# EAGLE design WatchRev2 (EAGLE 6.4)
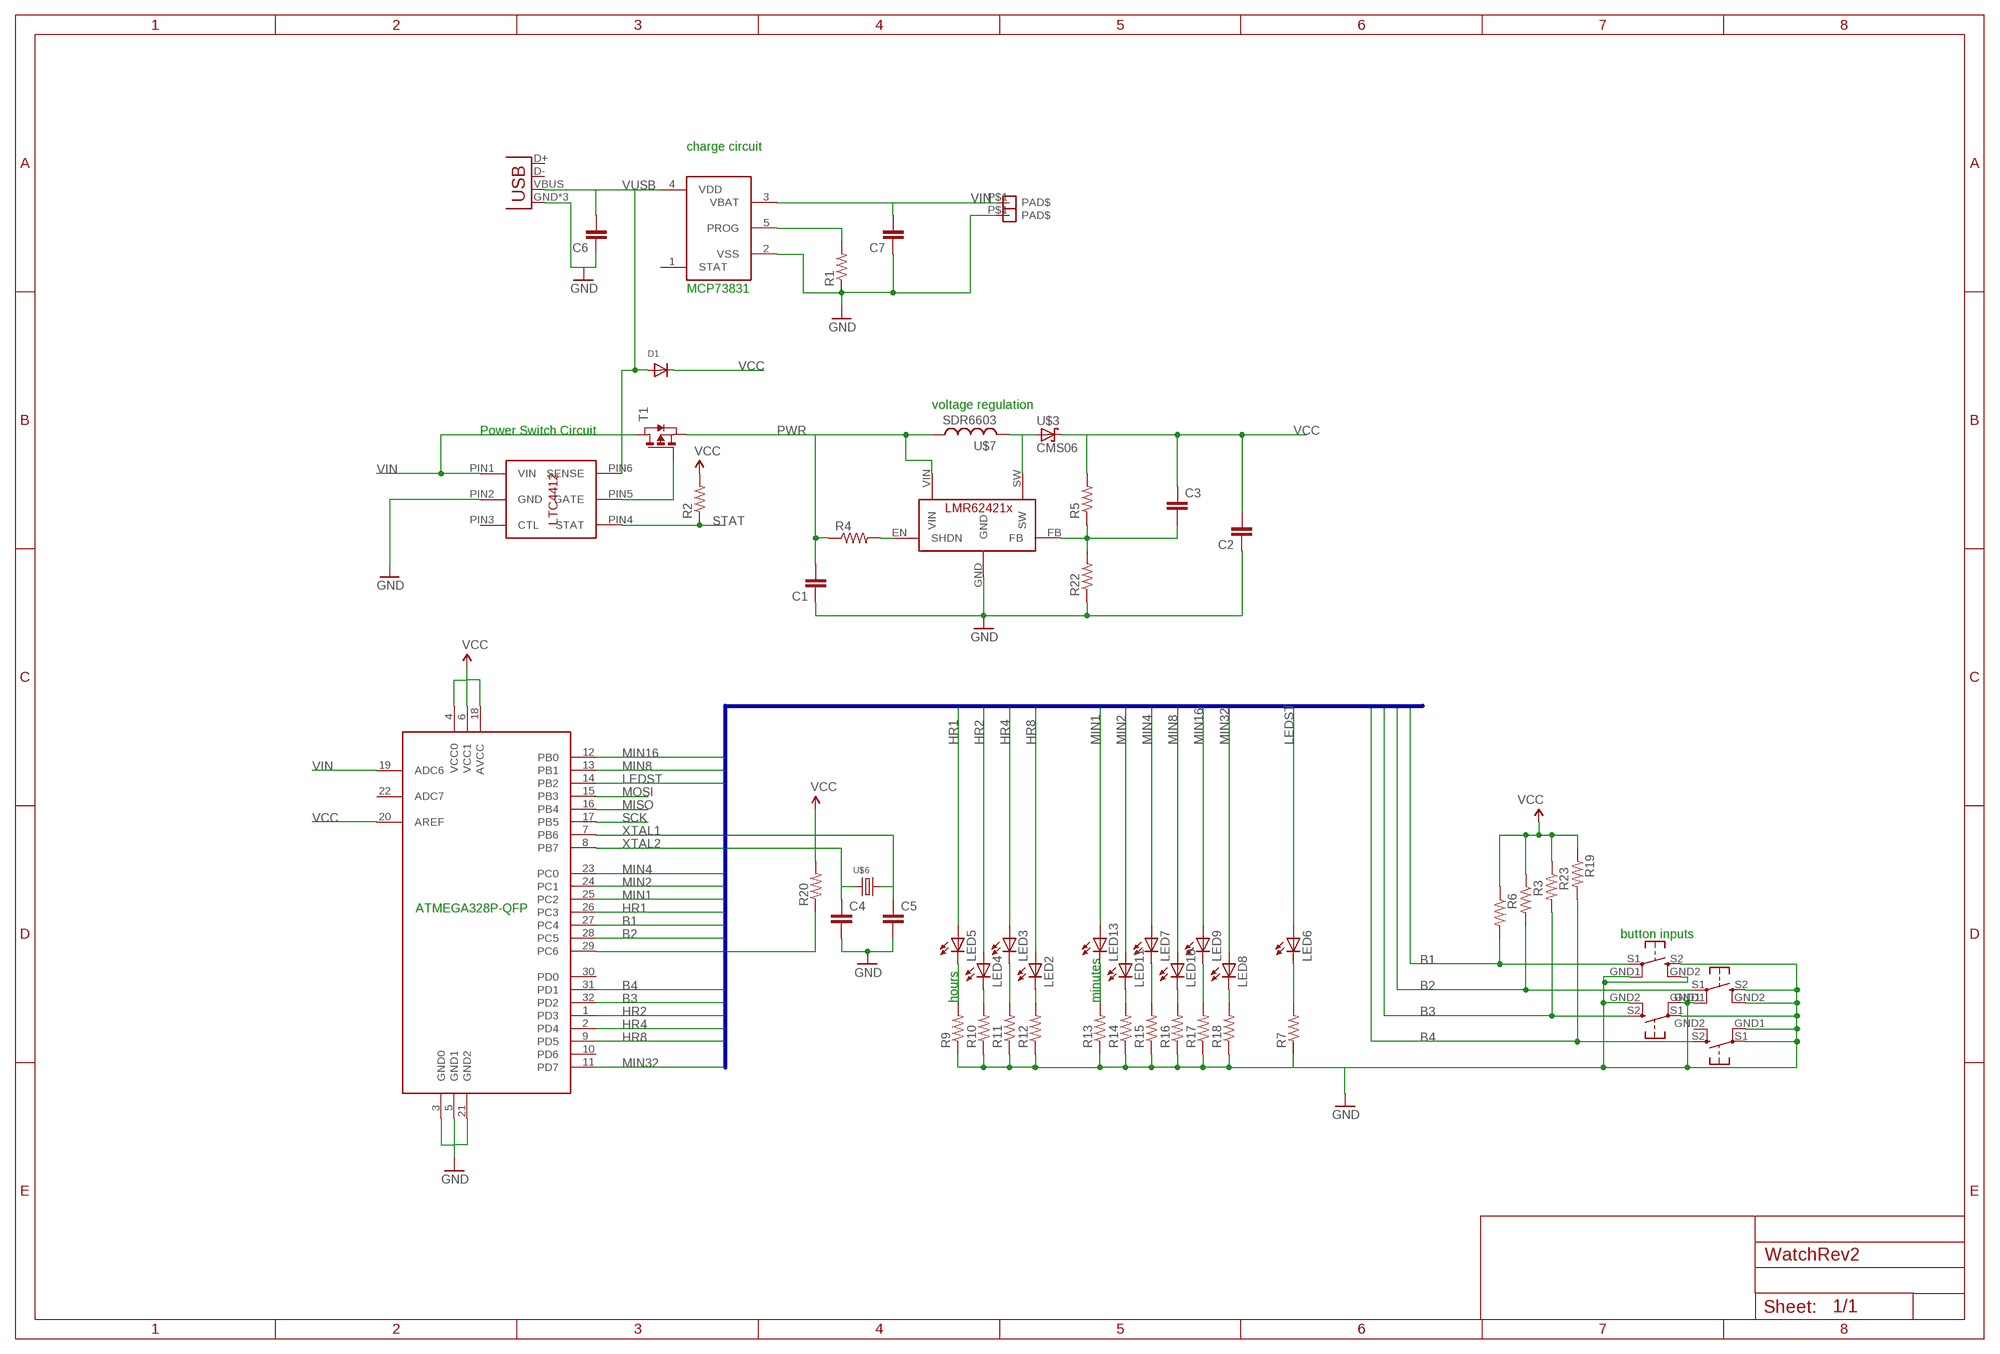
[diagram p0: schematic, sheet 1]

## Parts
C1  CAP0603-CAP  [0603-CAP]
C2  CAP0603-CAP  [0603-CAP]
C3  CAP0603-CAP  [0603-CAP]
C4  CAP0603-CAP  [0603-CAP]
C5  CAP0603-CAP  [0603-CAP]
C6  CAP0603-CAP  [0603-CAP]
C7  CAP0603-CAP  [0603-CAP]
D1  DIODESOD-123  [SOD-123]
JP5  USB-MICROB  [USB-MICROB]
LED2  LEDCHIPLED_1206  [CHIPLED_1206]
LED3  LEDCHIPLED_1206  [CHIPLED_1206]
LED4  LEDCHIPLED_1206  [CHIPLED_1206]
LED5  LEDCHIPLED_1206  [CHIPLED_1206]
LED6  LEDCHIPLED_0603  [CHIPLED_0603]
LED7  LEDCHIPLED_1206  [CHIPLED_1206]
LED8  LEDCHIPLED_1206  [CHIPLED_1206]
LED9  LEDCHIPLED_1206  [CHIPLED_1206]
LED10  LEDCHIPLED_1206  [CHIPLED_1206]
LED11  LEDCHIPLED_1206  [CHIPLED_1206]
LED13  LEDCHIPLED_1206  [CHIPLED_1206]
R1  RESISTOR0603-RES  [0603-RES]
R2  RESISTOR0603-RES  [0603-RES]
R3  RESISTOR0603-RES  [0603-RES]
R4  RESISTOR0603-RES  [0603-RES]
R5  RESISTOR0603-RES  [0603-RES]
R6  RESISTOR0603-RES  [0603-RES]
R7  RESISTOR0603-RES  [0603-RES]
R9  RESISTOR0603-RES  [0603-RES]
R10  RESISTOR0603-RES  [0603-RES]
R11  RESISTOR0603-RES  [0603-RES]
R12  RESISTOR0603-RES  [0603-RES]
R13  RESISTOR0603-RES  [0603-RES]
R14  RESISTOR0603-RES  [0603-RES]
R15  RESISTOR0603-RES  [0603-RES]
R16  RESISTOR0603-RES  [0603-RES]
R17  RESISTOR0603-RES  [0603-RES]
R18  RESISTOR0603-RES  [0603-RES]
R19  RESISTOR0603-RES  [0603-RES]
R20  RESISTOR0603-RES  [0603-RES]
R22  RESISTOR0603-RES  [0603-RES]
R23  RESISTOR0603-RES  [0603-RES]
T1  PMOSSOT23  [SOT-23]
U$1  ATMEGA328P  [TQFP32-08]
U$2  LMR62421X  [SOT-23_5PIN]
U$3  CMS06  [SOD-128]
U$4  MCP73831  [SOT-23_5GEN]
U$5  LTC4412  [LTC4412]
U$6  ECX-39  [ECX-39]
U$7  SDR6603  [SDR6603]
U$8  PAD  [PAD]
U$9  PAD  [PAD]
U$10  RA_TAC_BUTTON  [RA_TAC_BUTTON]
U$11  RA_TAC_BUTTON  [RA_TAC_BUTTON]
U$12  RA_TAC_BUTTON  [RA_TAC_BUTTON]
U$13  RA_TAC_BUTTON  [RA_TAC_BUTTON]

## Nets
B1: R6.2 U$1.27(PC4) U$10.S1
B2: R3.2 U$1.28(PC5) U$11.S1
B3: R23.2 U$1.32(PD2) U$12.S2
B4: R19.2 U$1.31(PD1) U$13.S2
GND: C1.1 C2.1 C4.2 C5.2 C6.1 C7.1 JP5.GND JP5.MT1(GND) JP5.MT2(GND) R1.1 R7.1 R9.1 R10.1 R11.1 R12.1 R13.1 R14.1 R15.1 R16.1 R17.1 R18.1 R22.1 U$1.3(GND0) U$1.5(GND1) U$1.21(GND2) U$2.GND U$4.2(VSS) U$5.PIN2(GND) U$9.P$1(PAD$) U$10.GND1 U$10.GND2 U$10.S2 U$11.GND1 U$11.GND2 U$11.S2 U$12.GND1 U$12.GND2 U$12.S1 U$13.GND1 U$13.S1
HR1: LED5.A U$1.26(PC3)
HR2: LED4.A U$1.1(PD3)
HR4: LED3.A U$1.2(PD4)
HR8: LED2.A U$1.9(PD5)
LEDST: LED6.A U$1.14(PB2)
MIN1: LED13.A U$1.25(PC2)
MIN2: LED11.A U$1.24(PC1)
MIN4: LED7.A U$1.23(PC0)
MIN8: LED10.A U$1.13(PB1)
MIN16: LED9.A U$1.12(PB0)
MIN32: LED8.A U$1.11(PD7)
MISO: U$1.16(PB4)
MOSI: U$1.15(PB3)
N$2: LED5.C R9.2
N$3: U$2.SW U$3.2(A) U$7.P$2
N$4: LED4.C R10.2
N$5: LED6.C R7.2
N$6: C3.2 R5.1 R22.2 U$2.FB
N$7: LED3.C R11.2
N$8: LED2.C R12.2
N$9: R4.2 U$2.EN(SHDN)
N$10: LED13.C R13.2
N$11: LED11.C R14.2
N$12: LED7.C R15.2
N$13: LED10.C R16.2
N$14: LED9.C R17.2
N$15: LED8.C R18.2
N$16: R20.1 U$1.29(PC6)
N$19: T1.3(G) U$5.PIN5(GATE)
N$21: R1.2 U$4.5(PROG)
PWR: C1.2 R4.1 T1.2(S) U$2.VIN U$7.P$1
SCK: U$1.17(PB5)
STAT: R2.1 U$5.PIN4(STAT)
VCC: C2.2 C3.1 D1.C R2.2 R3.1 R5.2 R6.1 R19.1 R20.2 R23.1 U$1.4(VCC0) U$1.6(VCC1) U$1.18(AVCC) U$1.20(AREF) U$3.1(C)
VIN: C7.2 T1.1(D) U$1.19(ADC6) U$4.3(VBAT) U$5.PIN1(VIN) U$8.P$1(PAD$)
VUSB: C6.2 D1.A JP5.VBUS U$4.4(VDD) U$5.PIN6(SENSE)
XTAL1: C5.1 U$1.7(PB6) U$6.P$2
XTAL2: C4.1 U$1.8(PB7) U$6.P$1
Unconnected: JP5.D+ JP5.D- U$1.10(PD6) U$1.22(ADC7) U$1.30(PD0) U$4.1(STAT) U$5.PIN3(CTL) U$13.GND2

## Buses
MIN32,MIN16,MIN8,MIN4,MIN2,MIN1,HR8,HR4,HR2,HR1,LEDST,B[1..4]

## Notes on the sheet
- charge circuit
- MCP73831
- voltage regulation
- Power Switch Circuit
- ATMEGA328P-QFP
- button inputs
- hours | minutes

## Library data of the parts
C1-C7 = SparkFun-Capacitors:CAP: Capacitor
D1 = adafruit:DIODE: Diode
JP5 = SparkFun-Connectors:USB: USB Connectors USB-B-PTH is fully proven SKU : PRT-00139/CONN-08278 USB-miniB is fully proven SKU : PRT-00587 USB-A-PCB is untested. USB-A-H is throughly reviewed, but untested. Spark Fun Electronics SKU : PRT-00437 USB-B-SMT is throughly reviewed, but untested. Needs silkscreen touching up.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; PROD_ID: CONN-09505
LED2-LED5 LED7-LED11 LED13 = adafruit:LED: LED
LED6 = led:LED: LED
R1-R7 R9-R20 R22 R23 = SparkFun-Passives:RESISTOR: Resistor
T1 = zetex:PMOSSOT23: MOS FET; OC_FARNELL: unknown; OC_NEWARK: unknown
U$1 = atmel:ATMEGA328P
U$2 = ubuntuMisc:LMR62421X
U$3 = ubuntuMisc:CMS06
U$4 = ubuntuMisc:MCP73831
U$5 = MyLibrary:LTC4412
U$6 = MyLibrary:ECX-39
U$7 = ubuntuMisc:SDR6603
U$8 U$9 = MyLibrary:PAD
U$10-U$13 = MyLibrary:RA_TAC_BUTTON

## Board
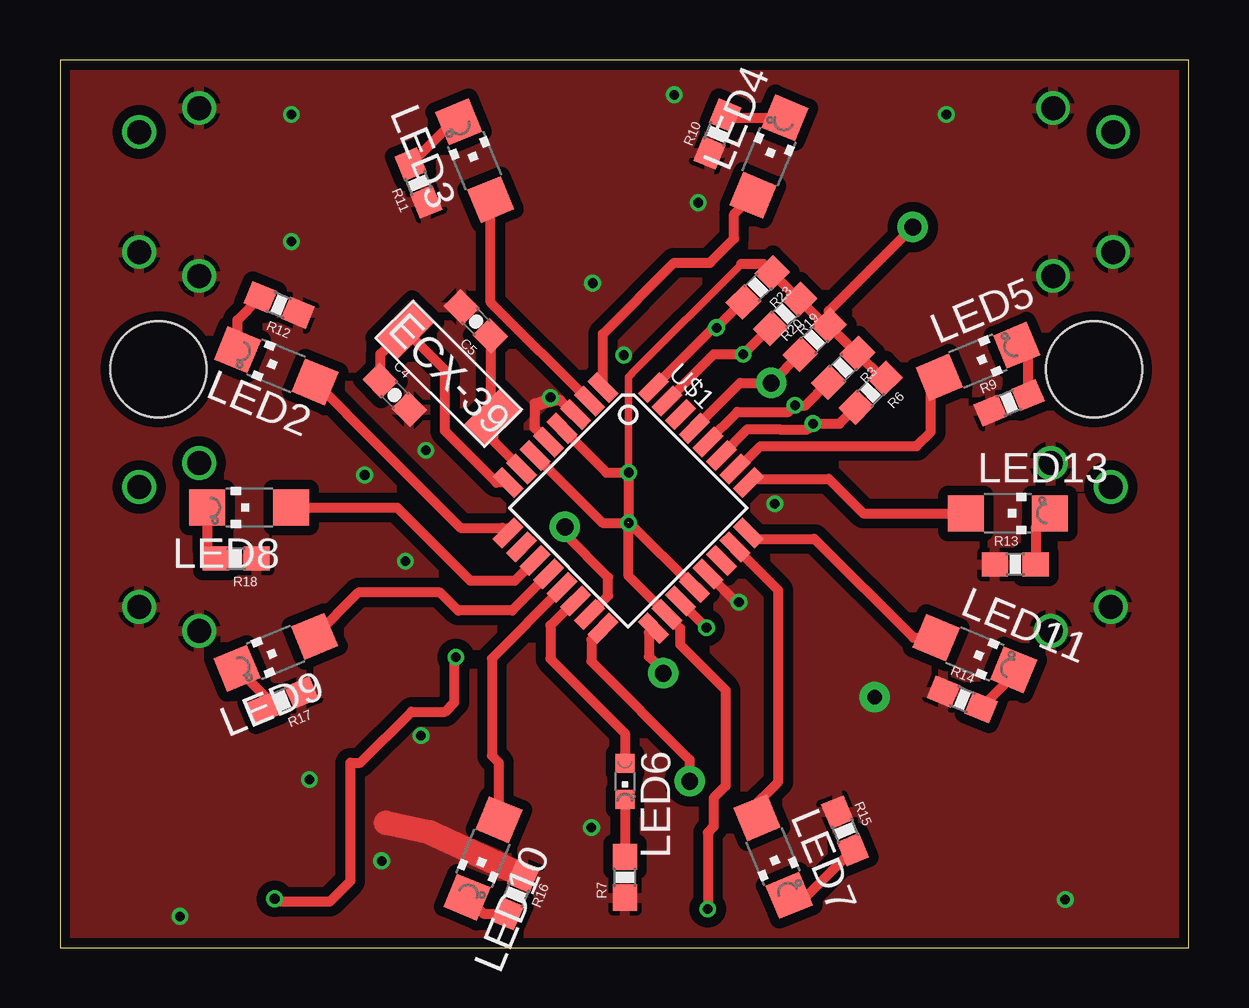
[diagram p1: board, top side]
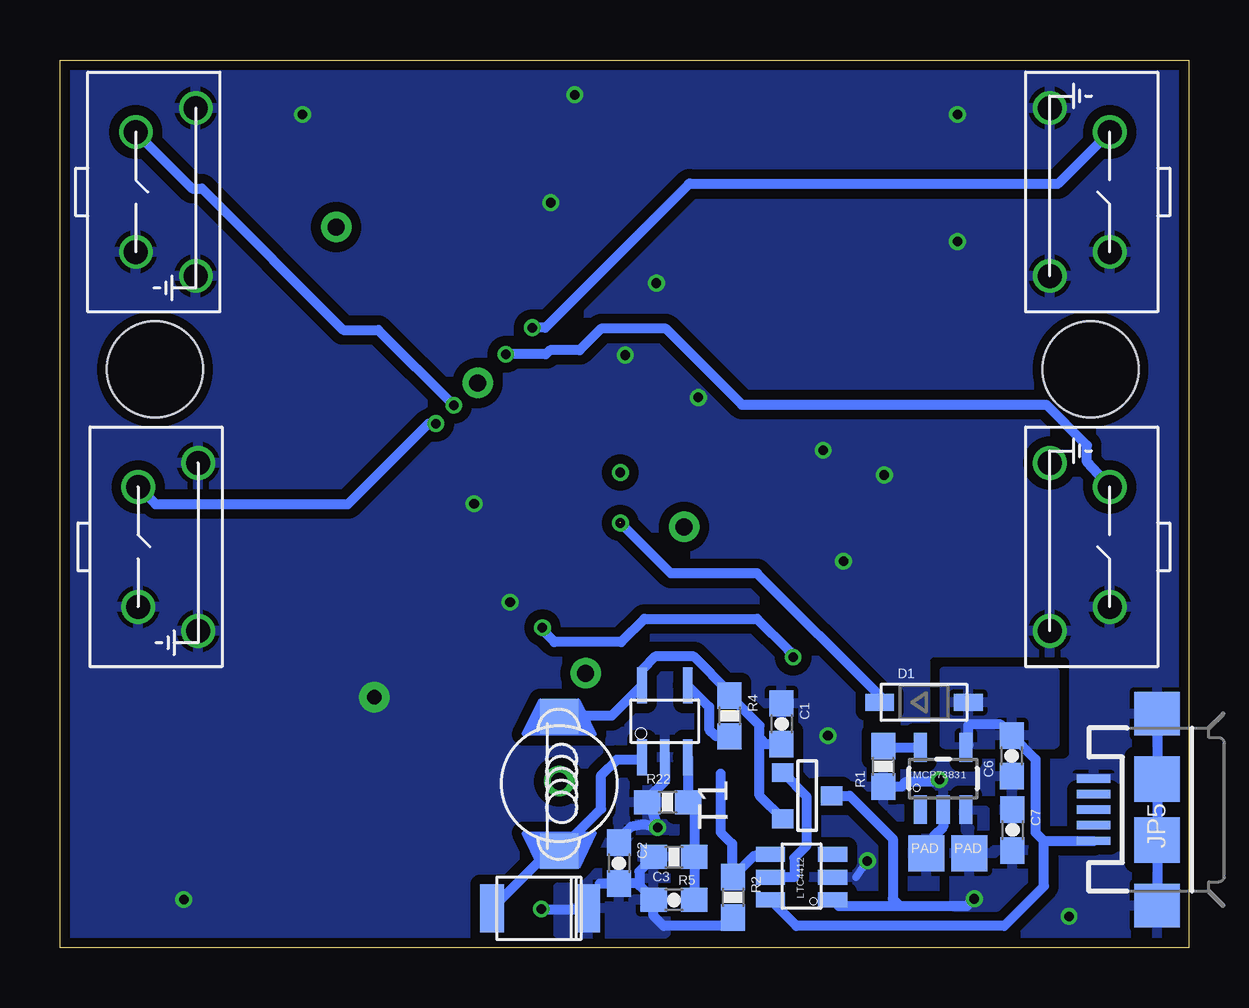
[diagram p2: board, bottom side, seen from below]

Size 47.06 x 37 mm. Coordinates in mm from the lower left corner, seen from the top.
Outline: 0,0 47.06,0 47.06,37 0,37 0,0
Copper layers (1*16): Top 0.035mm / dielectric 1.5mm / Bottom 0.035mm
Design rules "PCB-POOL Standard": minimum track width 0.15mm, minimum drill 0.3mm, track to track 0.15mm, track to pad 0.15mm, pad to pad 0.15mm, via to via 0.15mm, smd to smd 0.15mm, copper to edge 0.3mm, drill to drill 0.2mm, minimum pad ring 0.2mm, minimum via ring 0.15mm, stop-mask expansion 0.075mm, vias tented up to drill 0mil, thermal gap 0.2mm
Holes 4 mm at 4.1,24.1 43.1,24.1

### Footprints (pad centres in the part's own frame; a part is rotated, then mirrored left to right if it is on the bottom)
0603-CAP = smd 1.1 x 1: 1 -0.85,0; 2 0.85,0
SOD-123 = smd 1.2 x 0.7: A 1.85,0; C -1.85,0
USB-MICROB = smd 0.35 x 1.4: D+ 0,2.65; D- -0.65,2.65; GND 1.3,2.65; ID 0.65,2.65; VBUS -1.3,2.65 | smd 1.8 x 1.9: MT1 -4,0; MT2 4,0 | smd 1.9 x 1.9: P$1 -1.27,0; P$2 1.27,0
CHIPLED_1206 = smd 1.5 x 1.5: A 0,-1.75; C 0,1.75
CHIPLED_0603 = smd 0.8 x 0.8: A 0,-0.75; C 0,0.75
0603-RES = smd 1.1 x 1: 1 -0.85,0; 2 0.85,0
SOT-23 = smd 0.787 x 0.889: 1 0.025,-1.016; 2 -0.94,1.016; 3 0.991,1.016
TQFP32-08 = smd 1.27 x 0.559: 1 -4.293,2.8; 2 -4.293,2; 3 -4.293,1.2; 4 -4.293,0.4; 5 -4.293,-0.4; 6 -4.293,-1.2; 7 -4.293,-2; 8 -4.293,-2.8; 17 4.293,-2.8; 18 4.293,-2; 19 4.293,-1.2; 20 4.293,-0.4; 21 4.293,0.4; 22 4.293,1.2; 23 4.293,2; 24 4.293,2.8 | smd 0.559 x 1.27: 9 -2.8,-4.293; 10 -2,-4.293; 11 -1.2,-4.293; 12 -0.4,-4.293; 13 0.4,-4.293; 14 1.2,-4.293; 15 2,-4.293; 16 2.8,-4.293; 25 2.8,4.293; 26 2,4.293; 27 1.2,4.293; 28 0.4,4.293; 29 -0.4,4.293; 30 -1.2,4.293; 31 -2,4.293; 32 -2.8,4.293
SOT-23_5PIN = smd 0.4 x 1.5: EN -0.95,-1.5; FB -0.95,1.5; GND 0,1.5; SW 0.95,1.5; VIN 0.95,-1.5
SOD-128 = smd 2 x 1: 1 0,2; 2 0,-2
SOT-23_5GEN = smd 0.55 x 1.2: 1 -0.95,-1.3; 2 0,-1.3; 3 0.95,-1.3; 4 0.95,1.3; 5 -0.95,1.3
LTC4412 = smd 0.62 x 1.22: PIN1 -0.95,-1.3; PIN2 0,-1.3; PIN3 0.95,-1.3; PIN4 0.95,1.3; PIN5 0,1.3; PIN6 -0.95,1.3
ECX-39 = smd 1.3 x 2.2: P$1 -2.6,0; P$2 2.6,0
SDR6603 = smd 1.45 x 1.6: P$1 -2.8,0; P$2 2.8,0
PAD = smd 1.5 x 1.5: P$1 0,0
RA_TAC_BUTTON = drill 1: GND1 -3.5,2.5; GND2 3.5,2.5; S1 -2.5,0; S2 2.5,0

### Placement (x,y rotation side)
C1  16.98,9.33 270 bottom
C2  23.76,3.52 270 bottom
C3  21.47,1.99 0 bottom
C4  13.96,23.03 315 top
C5  17.34,26.1 135 top
C6  7.39,7.99 90 bottom
C7  7.35,4.9 270 bottom
D1  11.04,10.22 0 bottom
JP5  1.32,5.75 90 bottom
LED2  9.01,24.25 67.5 top
LED3  17.29,32.8 22.5 top
LED4  29.56,32.97 337.5 top
LED5  38.27,24.44 292.5 top
LED6  23.55,6.93 180 top
LED7  29.73,3.79 202.5 top
LED8  7.89,18.34 90 top
LED9  8.99,12.31 112.5 top
LED10  17.63,3.71 157.5 top
LED11  38.14,12.25 247.5 top
LED13  39.51,18.1 270 top
R1  12.74,7.55 90 bottom
R2  19.01,2.09 270 bottom
R3  32.64,24.17 225 top
R4  19.14,9.65 270 bottom
R5  21.47,3.77 180 bottom
R6  33.79,23.13 225 top
R7  23.55,2.93 90 top
R9  39.56,22.71 22.5 top
R10  27.4,33.91 67.5 top
R11  14.94,31.87 112.5 top
R12  9.14,26.79 157.5 top
R13  39.82,15.98 0 top
R14  37.61,10.34 337.5 top
R15  32.72,4.86 292.5 top
R16  18.99,2.2 247.5 top
R17  9.29,10.3 202.5 top
R18  7.35,16.22 180 top
R19  30.22,26.42 225 top
R20  31.45,25.33 45 top
R22  21.73,6.06 0 bottom
R23  29.09,27.52 225 top
T1  15.91,6.3 90 bottom
U$1  23.69,18.33 315 top
U$2  21.85,9.43 180 bottom
U$3  27.05,1.63 270 bottom
U$4  10.24,7.05 0 bottom
U$5  16.15,2.93 90 bottom
U$6  16.21,23.92 315 top
U$7  26.25,6.83 270 bottom
U$8  9.15,3.93 0 bottom
U$9  10.95,3.93 0 bottom
U$10  43.8,16.7 270 bottom
U$11  43.9,31.5 270 bottom
U$12  3.3,31.5 90 bottom
U$13  3.3,16.7 90 bottom

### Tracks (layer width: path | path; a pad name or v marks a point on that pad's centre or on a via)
B1  (via drill 0.4)
  Top 0.406: U$1.27 28.66,21.61 29.98,21.61 29.99,21.6 31.15,21.6 v31.39,21.84 32.5,21.84 R6.2
  Bottom 0.406: v31.39,21.84 31.7,21.84 35.06,18.48 43.08,18.48 U$10.S1
B2  (via drill 0.4)
  Top 0.406: U$1.28 27,21.1 28.23,22.33 30.37,22.33 v30.64,22.6 31.08,22.6 R3.2
  Bottom 0.406: v30.64,22.6 33.79,25.75 35.25,25.75 41.14,31.64 41.54,31.64 U$11.S1
B3  (via drill 0.4)
  Top 0.406: U$1.32 27.24,25.84 v27.37,25.84 28.45,26.92 R23.2
  Bottom 0.406: 20.82,31.85 20.84,31.83 | 20.84,31.83 26.83,25.84 v27.37,25.84 | U$12.S2 5.47,31.83 20.84,31.83
B4  (via drill 0.4)
  Top 0.406: U$1.31 27.26,24.73 v28.48,24.73 29.57,25.82 R19.2
  Bottom 0.406: v28.48,24.73 26.8,24.73 26.63,24.9 25.4,24.9 24.5,25.8 21.8,25.8 18.63,22.63 5.95,22.63 4.25,20.93 4.25,20.25 U$13.S2
GND  (via drill 0.4, 0.6 pad 1.27)
  Top 0.406: 28.15,14.4 28.15,14.43 U$1.21 27.07,15.58 | U$1.5 19.8,21.65 19.8,22.68 v20.45,22.93 20.05,22.63 20.85,22.83 21.47,22.21 U$1.3
  Top 1.016: R16.1 15.4,4.8 13.6,5.2
  Bottom 0.305: 13.89,2.93 v13.41,3.61
  Bottom 0.406: JP5.MT2 JP5.MT1 | v10.4,7 10.5,6.9 11.8,6.9 12,6.7 R1.1 | U$2.GND 21.85,6.93 22.55,6.23 v22.15,5 22.72,5.13 23.25,5.03 23.76,4.52 C2.1 | U$4.2 10.24,5.04 10.65,4.63 10.65,4.23 U$9.P$1
  other vias: 23.5,24.7 25.6,35.55 26.6,31.05 22.2,27.7 12.7,19.7 14.4,16.1 28.3,14.4 29.8,18.5 5,1.3 41.9,2 33.96,10.44 15.05,8.83 15.25,20.73 9.65,29.43 9.65,34.73 36.95,34.73
  pour Top (isolate 0.406): -0.2,37.28 47.5,36.98 47.5,-0.3 -0.2,0
  pour Bottom (isolate 0.406, rank 3): -1,36.63 47.85,36.93 47.85,0.1 -1,-0.2
HR1
  Top 0.406: U$1.26 28.25,19.95 29.2,20.9 35.7,20.9 36.3,21.5 36.3,23.42 LED5.A
HR2
  Top 0.406: U$1.1 22.63,25.58 25.6,28.55 27.1,28.55 28.1,29.55 28.1,30.57 LED4.A
HR4
  Top 0.406: U$1.2 17.96,26.89 LED3.A
HR8
  Top 0.406: 18.67,17.48 U$1.9 18.44,17.5 16.7,17.5 11.91,22.29 11.91,22.3 LED2.A
LEDST
  Top 0.406: U$1.14 21.46,14.44 20.45,13.43 20.45,12.03 23.55,8.93 LED6.A
MIN1
  Top 0.406: U$1.25 28.85,19.53 32.05,19.53 33.48,18.1 LED13.A
MIN2
  Top 0.406: U$1.24 28.94,17.03 31.45,17.03 35.56,12.92 LED11.A
MIN4
  Top 0.406: U$1.23 29.95,14.89 29.95,6.92 28.75,5.72 LED7.A
MIN8
  Top 0.406: U$1.13 20.93,14.98 18,12.05 18,8 18.3,7.7 LED10.A
MIN16
  Top 0.406: U$1.12 18.85,14.05 16.6,14.05 15.85,14.8 12.43,14.8 LED9.A
MIN32
  Top 0.406: U$1.11 18.96,15.3 17.1,15.3 14.06,18.34 LED8.A
MISO  (via drill 0.7 pad 1.27)
  Top 0.406: U$1.16 22.15,12.83 22.15,11.93 26.25,7.83 v26.25,6.93
MOSI  (via drill 0.7 pad 1.27)
  Top 0.406: U$1.15 22.85,14.66 22.85,15.43 21.05,17.23 v21.05,17.53
N$2
  Top 0.406: LED5.C 40.35,24.64 R9.2
N$3
  Bottom 0.406: U$2.SW 22.9,7.83 23.85,7.83 24.5,7.18 24.5,5.78 U$7.P$2 26.65,4.03 U$3.2
N$4
  Top 0.406: R10.2 27.83,34.59 LED4.C
N$5
  Top 0.406: LED6.C R7.2
N$6
  Bottom 0.406: C3.2 R5.1 20.62,5.8 R22.2 20.88,7.91 U$2.FB
N$7
  Top 0.406: R11.2 16.38,34.42 LED3.C
N$8
  Top 0.406: LED2.C 7.4,26.16 R12.2
N$9
  Bottom 0.406: R4.2 19.7,8.8 20,9.1 20,10.04 U$2.EN
N$10
  Top 0.406: LED13.C 40.67,17.5 R13.2
N$11
  Top 0.406: R14.2 39.75,11.37 LED11.C
N$12
  Top 0.406: LED7.C 31.15,2.17 R15.2
N$13
  Top 0.406: LED10.C 17.65,1.41 R16.2
N$14
  Top 0.406: LED9.C 8.5,10.51 R17.2
N$15
  Top 0.406: LED8.C 6.14,16.57 R18.2
N$16  (via drill 0.7 pad 1.27)
  Top 0.406: U$1.29 26.46,21.65 28.35,23.53 v29.65,23.53 R20.1
N$19
  Bottom 0.406: T1.3 15.95,6.31 15.95,4.23 16.45,3.73 16.45,2.93 U$5.PIN5
N$21
  Bottom 0.406: R1.2 12.68,8.35 U$4.5
PWR
  Bottom 0.406: 17.9,8.73 17.9,6.33 T1.2 | 17.9,8.73 17.9,9.26 R4.1 19.14,10.64 20.63,12.13 22.25,12.13 22.8,11.58 U$2.VIN 24.07,9.66 26.22,9.66 U$7.P$1 | C1.2 17.65,8.48 17.9,8.73
SCK  (via drill 0.7 pad 1.27)
  Top 0.406: U$1.17 24.55,13.12 24.55,12.13 25.15,11.53 v25.15,11.43
STAT
  Bottom 0.305: U$5.PIN4 18.07,3.88 18.14,3.81
  Bottom 0.406: 18.92,2.86 R2.1 | 18.14,3.81 R2.1 | 19.52,7.25 19.52,4.8 19.05,4.33 19.05,2.98 R2.1
VCC  (via drill 0.4, 0.7 pad 1.27)  (1 unrouted)
  Top 0.305: v23.7,19.8 23.7,23.79 23.85,23.93 23.85,23.95 28.4,28.5
  Top 0.406: R6.1 34.28,23.73 R3.1 33.22,24.77 R20.2 | R20.2 31.91,25.93 R19.1 30.79,27.02 R23.1 29.31,28.5 28.4,28.5 | 23.7,17.75 v23.7,19.8 22.78,19.8 U$1.4 | U$1.6 22.62,17.7 v23.7,17.7 | v23.7,17.7 23.7,15.49 U$1.18 25.31,13.84 25.85,13.3 25.85,12.63 27.75,10.73 27.75,6.73 27.25,6.23 27.25,5.03 27,4.79 v27,1.6 | v35.55,30.03 32.05,26.54 R20.2 | U$1.20 23.75,17.7 v23.7,17.7
  Bottom 0.406: 23.93,2.5 C2.2 | 24.55,2.67 C2.2 | R2.2 19.35,0.9 21.9,0.9 22.32,1.32 C3.1 22.91,2.59 | 22.91,2.59 23,2.67 C2.2 | R5.2 22.91,3.18 22.91,2.59 | D1.C 12.89,10.49 18,15.6 21.6,15.6 v23.7,17.7 | v27,1.6 25.08,1.6 U$3.1
  pour Bottom: 21.8,0.6 21.8,4 22.8,4 22.8,3.5 23.2,3.1 24.7,3.1 25.3,2.5 26.3,2.5 26.3,0.6
VIN  (via drill 0.4)
  Top 0.406: 25.87,14.43 U$1.19 25.87,14.41 v26.95,13.33 | v8.95,2.03 9.07,1.91 11.25,1.91 12.1,2.76 12.1,7.7 12.51,7.7 14.65,9.83 16.05,9.83 16.45,10.23 16.45,12.05 v16.5,12.1
  Bottom 0.406: C7.2 7.57,3.83 | v16.5,12.1 16.7,12.4 18,13.7 22.7,13.7 23.67,12.73 26.45,12.73 26.95,13.23 v26.95,13.33 | U$5.PIN1 14.6,1.73 12.05,1.73 | 12.05,1.73 9.25,1.73 v8.95,2.03 | T1.1 14.14,6.33 12.35,4.53 12.35,2.03 12.05,1.73
  pour Bottom: 9.8,1.7 8,1.7 6.9,2.8 6.9,4.2 8.5,4.2 8.5,5.7 9.4,5.7 9.4,4.4 9.8,4.4
VUSB
  Bottom 0.305: U$5.PIN6 17.32,1.98
  Bottom 0.406: 6.05,4.45 6.4,4.8 6.4,7.85 C6.2 7.85,9.3 9.19,9.3 9.19,8.45 U$4.4 | 6.05,4.45 JP5.VBUS | 6.05,4.45 6.05,2.55 7.7,0.9 16.36,0.9 U$5.PIN6
  pour Bottom (isolate 0.4, rank 2): 5.6,11.5 10.2,11.5 10.2,8.5 5.6,8.5
XTAL1
  Top 0.406: C5.1 17.94,22.18 U$6.P$2 18.04,21.14 U$1.7
XTAL2
  Top 0.406: C4.1 13.35,24.74 U$6.P$1 16.05,24.07 16.05,21.53 18.2,19.38 U$1.8

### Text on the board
tValues: MIN+ | SLEEP | HR+ | TIME | Designed by: | Nick Williams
